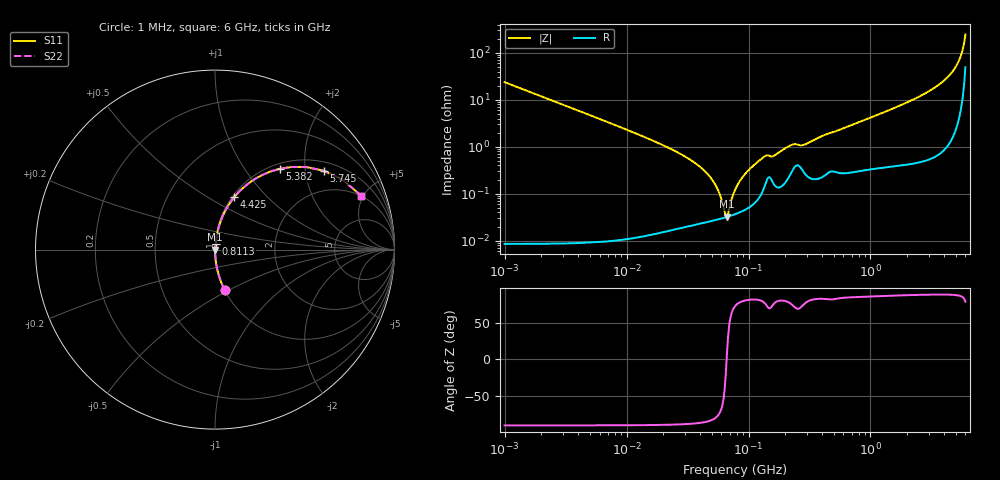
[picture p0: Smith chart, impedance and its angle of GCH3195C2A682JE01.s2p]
!Murata Part Number: GCH3195C2A682JE01
!These Parameters are Measured in Series Mode Connection
!Data Generated on Jun 19, 2026
!  o--ll--o
!Port1  Port2
!  o------o
!Operation Temp=25[degC], DC Bias Voltage=0[V]
!Freq. Start=1000[kHz] Stop=6[GHz] 401[Steps]
# Hz S RI R 50
!Freq.(Hz) S11(Real) S11(Imag) S21(Real) S21(Imag) S12(Real) S12(Imag) S22(Real) S22(Imag)
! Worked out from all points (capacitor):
!   401 points, 1 MHz to 6 GHz, reference 50 ohm
!   read as one part in series: C = 6.7 nF near 1.044 MHz
!   lowest |Z| = 32.4 mohm at 66.52 MHz (marker M1)
!   series resonance near 66.15 MHz, so ESL is about 860 pH
!   S11 on the Smith chart (normalised r, x): 1 MHz: 1.00, -0.47; 811.3 MHz: 1.01, +0.07; 4.425 GHz: 1.02, +0.66; 5.382 GHz: 1.09, +1.48; 5.745 GHz: 1.26, +2.53; 6 GHz: 1.98, +4.82
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1000000  0.0535 -0.2248  0.9465 0.2248  0.9465 0.2248  0.0535 -0.2248
4293785  0.00311 -0.0549  0.9969 0.0549  0.9969 0.0549  0.00311 -0.0549
1.843659e7  0.000285 -0.0118  0.9997 0.0118  0.9997 0.0118  0.000285 -0.0118
3.175522e7  0.000234 -0.00572  0.9998 0.00572  0.9998 0.00572  0.000234 -0.00572
4.497189e7  0.000255 -0.00282  0.9997 0.00282  0.9997 0.00282  0.000255 -0.00282
5.469524e7  0.000281 -0.00137  0.9997 0.00137  0.9997 0.00137  0.000281 -0.00137
6.368941e7  0.000311 -0.000271  0.9997 0.000271  0.9997 0.000271  0.000311 -0.000271
6.652088e7  0.000321 4.05e-05  0.9997 -4.05e-05  0.9997 -4.05e-05  0.000321 4.05e-05
7.745967e7  0.000368 0.00114  0.9996 -0.00114  0.9996 -0.00114  0.000368 0.00114
9.420718e7  0.000466 0.00264  0.9995 -0.00264  0.9995 -0.00264  0.000466 0.00264
1.334167e8  0.00133 0.00591  0.9987 -0.00591  0.9987 -0.00591  0.00133 0.00591
1.622626e8  0.0016 0.00627  0.9984 -0.00627  0.9984 -0.00627  0.0016 0.00627
2.248532e8  0.00295 0.0105  0.9971 -0.0105  0.9971 -0.0105  0.00295 0.0105
3.325952e8  0.00224 0.0132  0.9978 -0.0132  0.9978 -0.0132  0.00224 0.0132
8.112906e8  0.00414 0.0334  0.9959 -0.0334  0.9959 -0.0334  0.00414 0.0334
1.428092e9  0.00731 0.0598  0.9927 -0.0598  0.9927 -0.0598  0.00731 0.0598
2.927209e9  0.0256 0.1412  0.9744 -0.1412  0.9744 -0.1412  0.0256 0.1412
4.425027e9  0.1065 0.2913  0.8935 -0.2913  0.8935 -0.2913  0.1065 0.2913
4.93336e9  0.1954 0.3754  0.8046 -0.3754  0.8046 -0.3754  0.1954 0.3754
5.38176e9  0.3616 0.4504  0.6384 -0.4504  0.6384 -0.4504  0.3616 0.4504
5.744609e9  0.6065 0.4393  0.3935 -0.4393  0.3935 -0.4393  0.6065 0.4393
6e9  0.8141 0.3001  0.1859 -0.3001  0.1859 -0.3001  0.8141 0.3001
